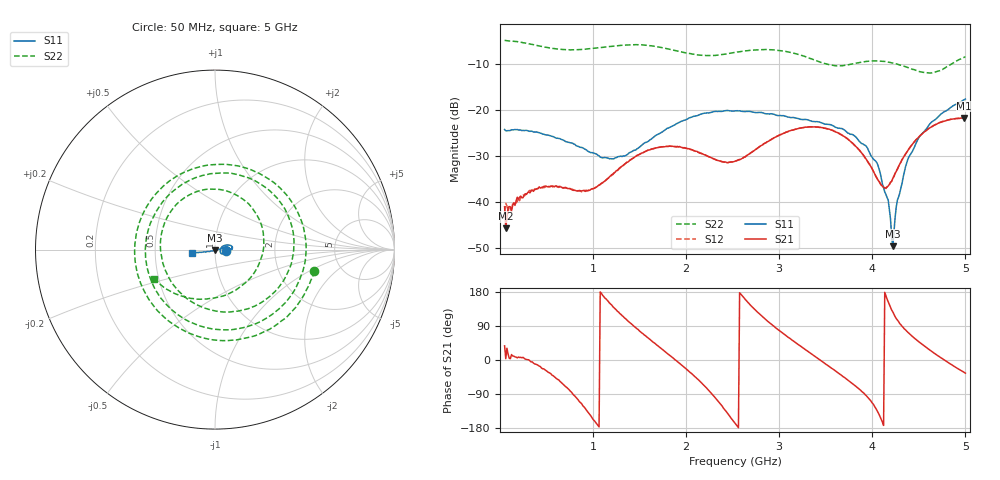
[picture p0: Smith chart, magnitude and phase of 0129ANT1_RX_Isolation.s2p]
! MASWSS0129 de-embedded Sparameters using port extention method. ANT1 to RX Isolation using 3 volt control
! 100pF blocking capacitor
! Sample board 1000013136
# Hz  S  DB  R  50
! Freq  S11  S21  S12  S22
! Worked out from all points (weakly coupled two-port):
!   401 points, 50 MHz to 5 GHz, reference 50 ohm
!   highest |S21| = -21.80 dB at 4.988 GHz (marker M1); lowest = -45.7 dB at 62.38 MHz (marker M2)
!   lowest |S11| = -49.6 dB at 4.22 GHz (marker M3), VSWR 1.01, Z = 50 - j0.332 ohm
!   |S11| at or under -10 dB: start of sweep to end of sweep
!   |S22| runs from -12.0 to -5.0 dB; largest |S21 - S12| = 0.0094
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5e7  -24.27 -5.1  -41.05 37.3  -42.07 -30.3  -4.97 -12.2
6.2375e7  -24.56 -3.8  -45.70 3.5  -40.28 15.0  -4.97 -15.3
4.08875e8  -24.92 -20.7  -37.11 -13.9  -37.03 -16.3  -6.10 -98.4
6.44e8  -26.26 -30.3  -36.71 -56.3  -36.57 -54.6  -6.88 -158.8
8.79125e8  -28.18 -32.5  -37.62 -115.8  -37.80 -115.2  -6.90 141.5
1.139e9  -30.38 -15.0  -35.22 161.2  -35.30 161.1  -6.37 79.5
1.39888e9  -29.24 12.5  -30.87 97.9  -30.89 97.9  -5.91 20.7
1.70825e9  -25.23 24.5  -28.17 35.1  -28.15 34.9  -6.40 -52.0
1.90625e9  -22.94 20.9  -27.97 -4.3  -27.98 -4.5  -7.26 -101.0
2.14138e9  -21.10 14.7  -29.36 -54.5  -29.25 -54.7  -8.14 -162.7
2.525e9  -20.25 5.2  -31.14 -166.5  -31.09 -166.8  -7.55 99.4
2.95813e9  -21.09 1.4  -25.95 85.6  -25.92 85.5  -7.05 9.7
3.35413e9  -22.53 9.4  -23.69 14.4  -23.72 14.5  -9.01 -79.1
3.65113e9  -24.00 13.1  -25.22 -37.3  -25.23 -37.6  -10.46 -164.8
3.93575e9  -27.92 9.9  -30.75 -94.4  -30.83 -94.5  -9.51 122.5
4.18325e9  -41.62 -23.2  -36.20 146.1  -36.20 145.4  -9.71 69.9
4.22038e9  -49.58 -86.7  -34.88 127.0  -34.79 125.7  -9.86 61.4
4.3565e9  -32.39 -161.3  -29.59 79.5  -29.62 79.0  -10.66 28.5
4.49263e9  -26.30 -166.3  -26.04 49.6  -26.04 49.4  -11.62 -9.7
4.74013e9  -20.88 -170.2  -22.70 5.4  -22.62 4.9  -11.35 -91.9
4.98763e9  -17.81 -172.9  -21.80 -32.7  -21.81 -33.3  -8.61 -152.4
5e9  -17.68 -172.7  -21.80 -34.8  -21.82 -35.3  -8.49 -154.4
